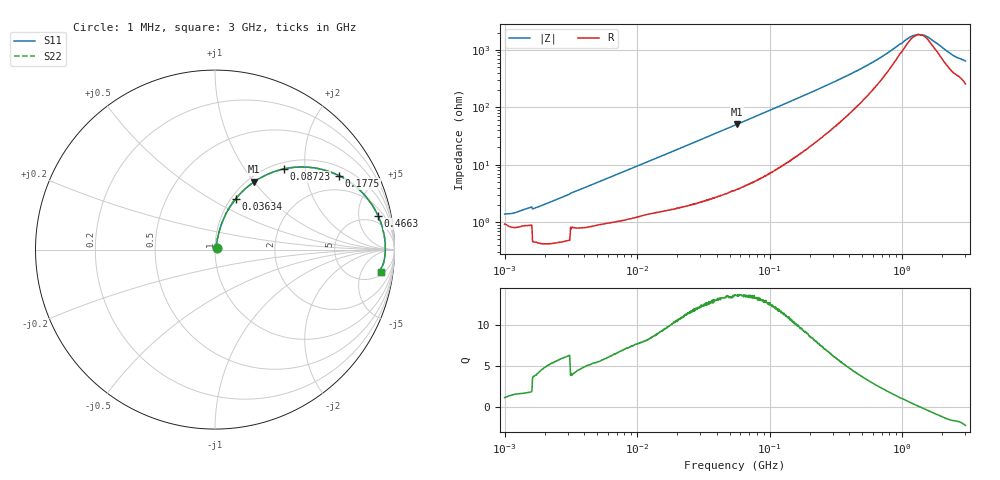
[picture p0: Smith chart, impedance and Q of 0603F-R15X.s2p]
!s-Parameter Generated by FASTRON Sdn. Bhd.
!FASTRON P/N : 0603F-R15X
!Keysight Technologies: E4991B_MY54100416_A.01.15
!Date: Thu Jun 20 13:07:59 2024
!Version  :Rev00  Thu Jun 20 13:07:59 2024
!Data & Calibration Information:
!Freq  S11  S21  S12  S22
!PortZ  Port1:50+j0  Port2:50+j0
!When reading reference impedance value at option line is always used.
! Remarks : This data is being provided solely for informational purposes.
# Hz S dB R 50
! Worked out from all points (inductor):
!   1601 points, 1 MHz to 3 GHz, reference 50 ohm
!   read as one part in series: L = 161 nH near 1.041 MHz
!   highest Q = 13.6 at 56.44 MHz (marker M1), where L = 141 nH
!   self-resonance near 1.349 GHz
!   S11 on the Smith chart (normalised r, x): 1 MHz: 1.02, +0.02; 36.34 MHz: 1.05, +0.66; 87.23 MHz: 1.12, +1.54; 177.5 MHz: 1.33, +3.12; 466.3 MHz: 3.17, +8.60; 3 GHz: 6, -12
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1000000  -37.30 47.4  -0.08 -0.6  -0.08 -0.6  -37.30 47.4
1173660  -36.90 55.4  -0.07 -0.7  -0.07 -0.7  -36.90 55.4
1545498  -35.00 59.6  -0.08 -0.9  -0.08 -0.9  -35.00 59.6
1691165  -35.20 74.2  -0.04 -1.0  -0.04 -1.0  -35.20 74.2
3804036  -28.50 75.8  -0.07 -2.1  -0.07 -2.1  -28.50 75.8
1.447069e7  -17.60 76.1  -0.20 -7.5  -0.20 -7.5  -17.60 76.1
2.422863e7  -13.50 72.8  -0.36 -12.2  -0.36 -12.2  -13.50 72.8
3.633776e7  -10.30 67.9  -0.64 -17.6  -0.64 -17.6  -10.30 67.9
5.504702e7  -7.37 60.5  -1.18 -25.3  -1.18 -25.3  -7.37 60.5
5.644167e7  -7.20 60.0  -1.23 -25.8  -1.23 -25.8  -7.20 60.0
8.723049e7  -4.59 49.6  -2.34 -36.0  -2.34 -36.0  -4.59 49.6
1.225874e8  -3.04 40.5  -3.72 -44.6  -3.72 -44.6  -3.04 40.5
1.775263e8  -1.88 30.7  -5.79 -53.2  -5.79 -53.2  -1.88 30.7
2.083556e8  -1.53 26.8  -6.86 -56.4  -6.86 -56.4  -1.53 26.8
3.047674e8  -0.97 18.7  -9.75 -62.0  -9.75 -62.0  -0.97 18.7
4.66327e8  -0.65 11.7  -13.60 -64.1  -13.60 -64.1  -0.65 11.7
7.925923e8  -0.49 5.2  -19.70 -55.7  -19.70 -55.7  -0.49 5.2
1.159346e9  -0.46 1.4  -25.00 -24.4  -25.00 -24.4  -0.46 1.4
1.367504e9  -0.46 -0.1  -25.70 2.2  -25.70 2.2  -0.46 -0.1
1.54974e9  -0.46 -1.3  -25.00 22.7  -25.00 22.7  -0.46 -1.3
2.41921e9  -0.58 -5.8  -18.60 53.8  -18.60 53.8  -0.58 -5.8
3e9  -0.60 -7.7  -16.70 58.8  -16.70 58.8  -0.60 -7.7
